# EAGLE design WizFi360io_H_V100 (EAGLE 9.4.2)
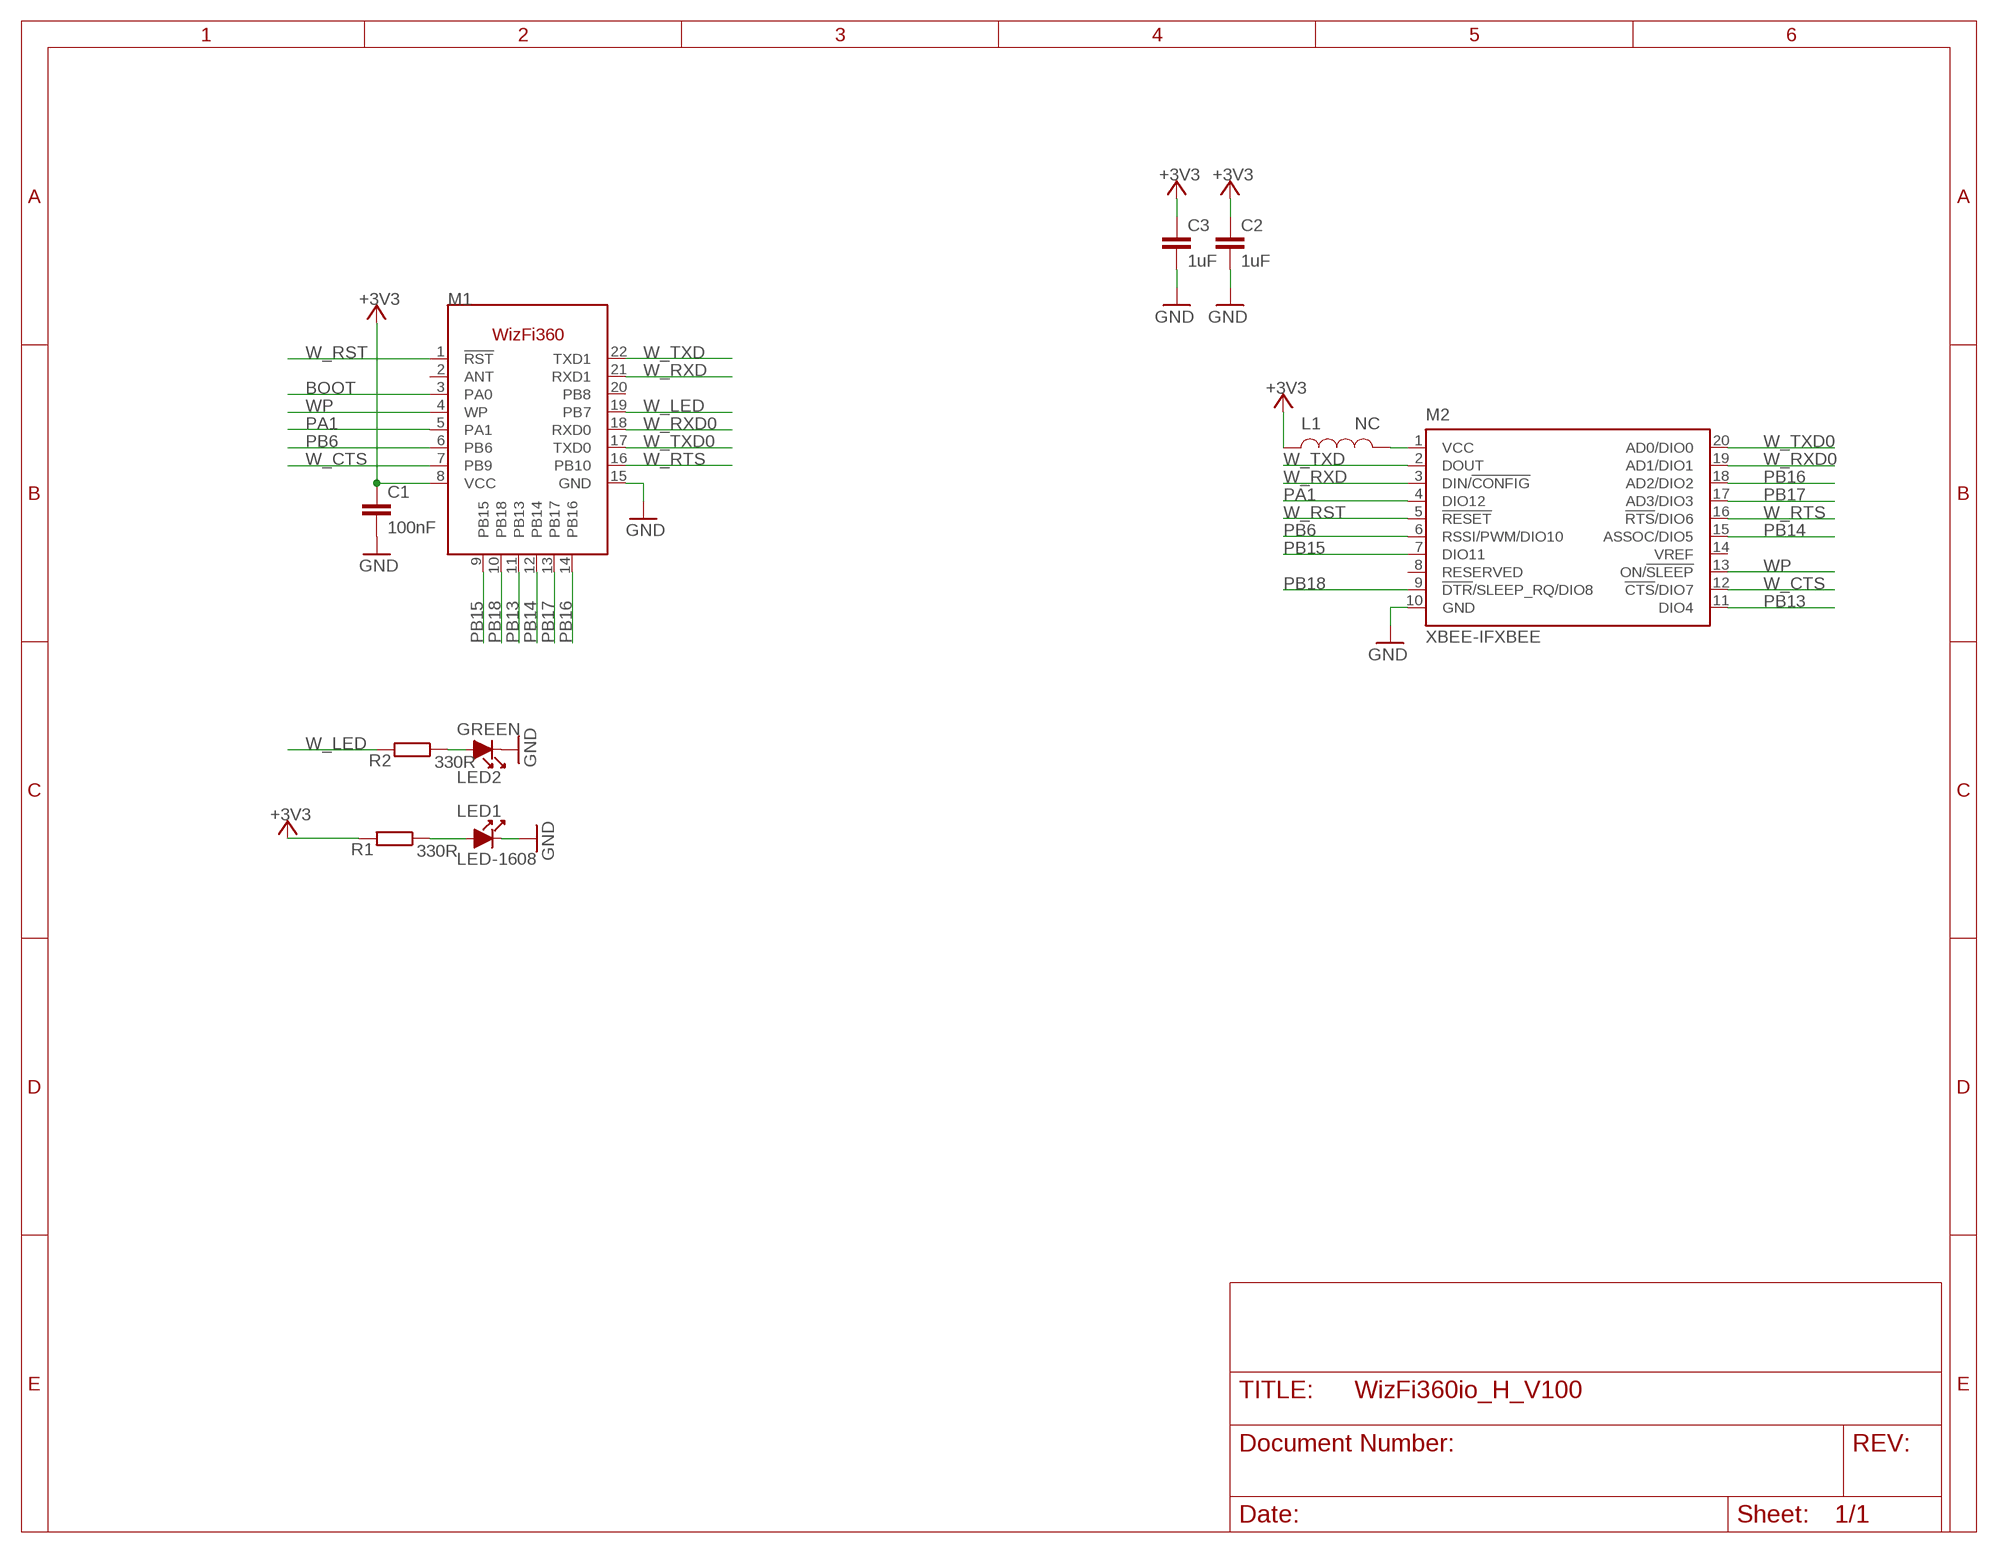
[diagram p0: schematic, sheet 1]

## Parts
C1  100nF  0142_10NF_0603  [C0603-ROUND@1]
C2  1uF  0142_10NF_0603  [C0603-ROUND@1]
C3  1uF  0142_10NF_0603  [C0603-ROUND@1]
L1  NC  L-1608  [L-1608]
LED1  LED-1608  [LED-1608]
LED2  GREEN  LED-1608  [LED-1608]
M1  WIZFI360  [WIZFI360]
M2  XBEE-IFXBEE  [XBEE-IF]
R1  330R  0028_CR0603JW103L  [R0603-ROUND]
R2  330R  0028_CR0603JW103L  [R0603-ROUND]

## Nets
+3V3 [power]: C1.1 C2.1 C3.1 L1.1 M1.8(VCC) R1.2
BOOT: M1.3(PA0)
GND: C1.2 C2.2 C3.2 LED1.K LED2.K M1.15(GND) M2.10(GND)
N$1: L1.P$2 M2.1(VCC)
N$7: LED1.A R1.1
N$17: LED2.A R2.1
PA1: M1.5(PA1) M2.4(DIO12)
PB6: M1.6(PB6) M2.6(RSSI/PWM/DIO10)
PB13: M1.11(PB13) M2.11(DIO4)
PB14: M1.12(PB14) M2.15(ASSOC/DIO5)
PB15: M1.9(PB15) M2.7(DIO11)
PB16: M1.14(PB16) M2.18(AD2/DIO2)
PB17: M1.13(PB17) M2.17(AD3/DIO3)
PB18: M1.10(PB18) M2.9(!DTR!/SLEEP_RQ/DIO8)
W_CTS: M1.7(PB9) M2.12(!CTS!/DIO7)
W_LED: M1.19(PB7) R2.2
W_RST: M1.1(!RST!) M2.5(!RESET)
W_RTS: M1.16(PB10) M2.16(!RTS!/DIO6)
W_RXD: M1.21(RXD1) M2.3(DIN/!CONFIG)
W_RXD0: M1.18(RXD0) M2.19(AD1/DIO1)
W_TXD: M1.22(TXD1) M2.2(DOUT)
W_TXD0: M1.17(TXD0) M2.20(AD0/DIO0)
WP: M1.4(WP) M2.13(ON/!SLEEP)
Unconnected: M1.2(ANT) M1.20(PB8) M2.8(RESERVED) M2.14(VREF)

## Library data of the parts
C1-C3 = Condensatori:0142_10NF_0603: 10nF 0603; CASE: 0603; MONTHLY_USAGE: _____; PART_NUMBER: 10nF_0603; PRICE: _____; SUPPLIER: _____; TYPE: Condensatori; VALUE: 10nF
L1 = INDUCTOR:L-1608
LED1 LED2 = DIODE:LED-1608
M1 = WIZnet:WIZFI360
M2 = xbee:XBEE-IF
R1 R2 = Resistenze:0028_CR0603JW103L: 10K 0603; CASE: 0603; MONTHLY_USAGE: _____; PART_NUMBER: CR0603JW103L; PRICE: _____; SUPPLIER: _____; TYPE: Resistenze; VALUE: 10k

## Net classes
0 default: width 0.203 mm, drill 0.008 mm, clearance 0.127 mm
1 power: width 0.305 mm, drill 0.3 mm, clearance 0.203 mm

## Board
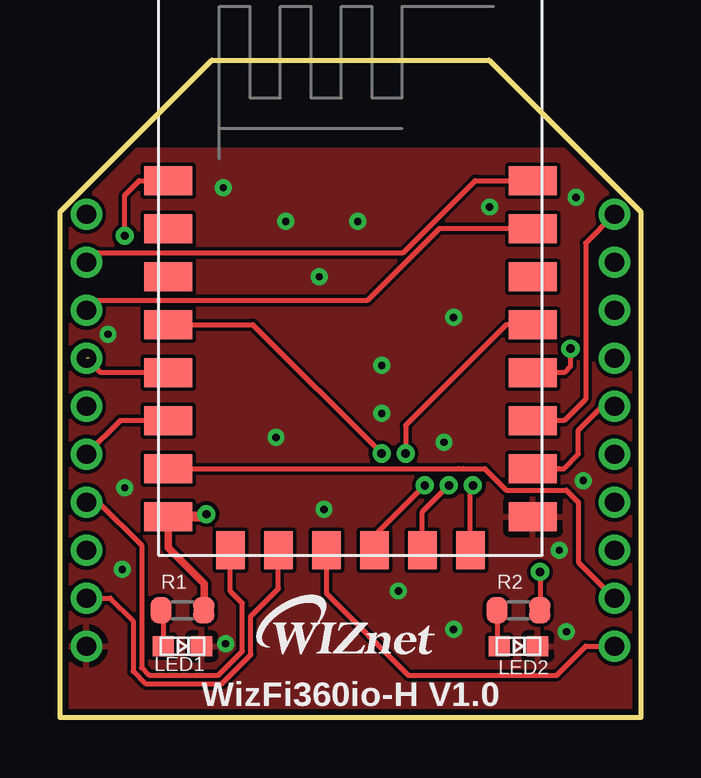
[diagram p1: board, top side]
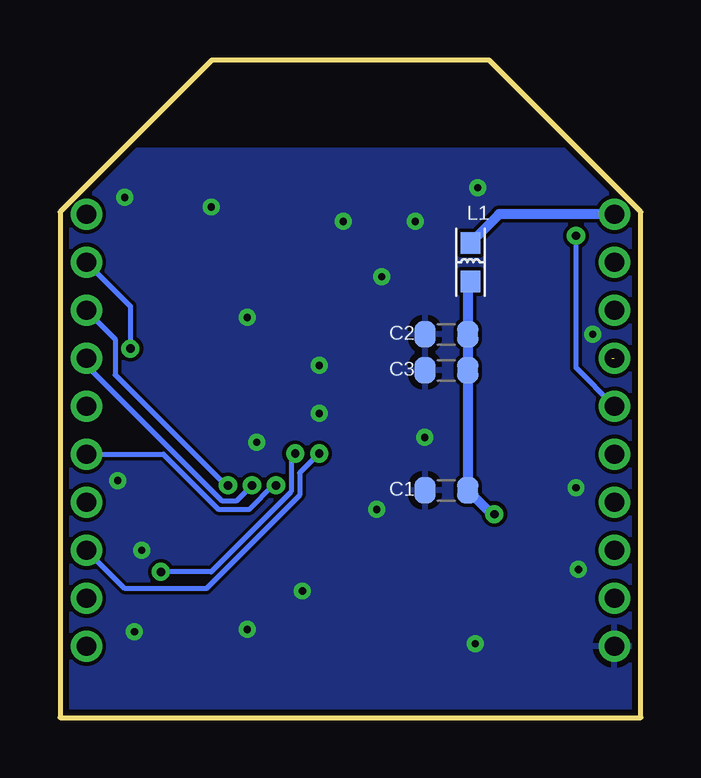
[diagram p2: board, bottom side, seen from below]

Size 24.2 x 27.4 mm. Coordinates in mm from the lower left corner, seen from the top.
Copper layers (1*16): Top 0.035mm / dielectric 1.5mm / Bottom 0.035mm
Design rules "default *": minimum track width 6mil, minimum drill 0.35mm, track to track 6mil, track to pad 6mil, pad to pad 6mil, via to via 6mil, smd to smd 6mil, copper to edge 10mil, drill to drill 10mil, minimum pad ring 10mil, minimum via ring 8mil, stop-mask expansion 4mil, vias tented up to drill 15mil, thermal gap 10mil

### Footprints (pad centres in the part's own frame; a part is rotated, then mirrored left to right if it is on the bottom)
C0603-ROUND@1 = smd 0.898 x 1.1: 1 -0.889,0; 2 0.889,0
L-1608 = smd 0.89 x 0.82: 1 -0.8,0; P$2 0.8,0
LED-1608 = smd 0.89 x 0.82: A -0.8,0; K 0.8,0
WIZFI360 = smd 2 x 1.2: 1 -7.6,3.6; 2 -7.6,1.6; 3 -7.6,-0.4; 4 -7.6,-2.4; 5 -7.6,-4.4; 6 -7.6,-6.4; 7 -7.6,-8.4; 8 -7.6,-10.4; 15 7.6,-10.4; 16 7.6,-8.4; 17 7.6,-6.4; 18 7.6,-4.4; 19 7.6,-2.4; 20 7.6,-0.4; 21 7.6,1.6; 22 7.6,3.6 | smd 1.2 x 1.6: 9 -5,-11.8; 10 -3,-11.8; 11 -1,-11.8; 12 1,-11.8; 13 3,-11.8; 14 5,-11.8
XBEE-IF = drill 0.8 pad 1.27: 1 -11,9; 2 -11,7; 3 -11,5; 4 -11,3; 5 -11,1; 6 -11,-1; 7 -11,-3; 8 -11,-5; 9 -11,-7; 10 -11,-9; 11 11,-9; 12 11,-7; 13 11,-5; 14 11,-3; 15 11,-1; 16 11,1; 17 11,3; 18 11,5; 19 11,7; 20 11,9
R0603-ROUND = smd 0.898 x 1.1: 1 -0.889,0; 2 0.889,0

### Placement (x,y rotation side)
C1  8.1,9.47 180 bottom
C2  8.1,15.97 180 bottom
C3  8.1,14.47 180 bottom
L1  7.1,18.98 90 bottom
LED1  5.1,2.97 0 top
LED2  19.1,2.97 0 top
M1  12.1,18.77 0 top
M2  12.1,11.97 0 top
R1  5.1,4.47 0 top
R2  19.1,4.47 0 top
U$1  [WIZNET3-LOGO]  8,2.62 0 top

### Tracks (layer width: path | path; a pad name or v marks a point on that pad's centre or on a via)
+3V3  (via drill 0.35)
  Top 0.305: M1.8 4.5,7.07 6,5.57 R1.2
  Top 0.406: v6.1,8.47 6,8.38 M1.8
  Bottom 0.406: L1.1 7.21,18.06 C2.1 C3.1 C1.1 6.21,8.47 v6.1,8.47
GND  (via drill 0.3)
  other vias: 14.1,5.27 6.9,3.07 20.8,6.97 21.1,3.57 13.4,12.67 16,11.47 9,11.67 10.8,18.38 17.9,21.27 21.5,21.67 6.8,22.08 2.7,9.57 2.6,6.17 11,8.67 13.4,14.67 16.4,16.67 12.4,20.67 9.4,20.67 16.4,3.67 21.8,9.88 2,15.97
  pour Top: -0.9,-1.03 25.1,-1.03 25.1,27.98 -0.9,27.98
  pour Bottom: -1.9,-2.03 26.1,-2.03 26.1,28.98 -1.9,28.98
N$1
  Bottom 0.406: M2.1 5.9,20.98 L1.P$2
N$7
  Top 0.203: R1.1 4.3,4.39 LED1.A
N$17
  Top 0.203: R2.1 18.21,3.06 LED2.A
PA1  (1 unrouted)
  Top 0.203: M1.5 1.7,14.38 1.22,14.86 1.22,14.97
PB6
  Top 0.203: M1.6 2.5,12.38 M2.6
PB13
  Top 0.203: M1.11 11.1,5.17 14.5,1.77 20.7,1.77 21.9,2.97 M2.11
PB14  (via drill 0.35)
  Top 0.203: M1.12 13.1,7.57 v15.2,9.67
  Bottom 0.203: M2.15 19.9,10.97 17.61,8.69 16.29,8.69 15.31,9.67 v15.2,9.67
PB15
  Top 0.203: M2.7 1.6,8.97 3.4,7.17 3.4,2.07 3.7,1.77 6.6,1.77 7.6,2.77 7.6,4.77 7.1,5.27 M1.9
PB16  (via drill 0.35)
  Top 0.203: M1.14 17.1,9.57 v17.2,9.67
  Bottom 0.203: M2.18 21.9,15.78 21.9,14.28 17.3,9.67 v17.2,9.67
PB17  (via drill 0.35)
  Top 0.203: M1.13 15.1,8.57 v16.2,9.67
  Bottom 0.203: M2.17 23.1,14.68 17.46,9.04 16.83,9.04 v16.2,9.67
PB18
  Top 0.203: M2.9 2.1,4.97 3.04,4.03 3.04,1.93 3.55,1.42 6.75,1.42 7.96,2.63 7.96,4.23 9.1,5.38 M1.10
W_CTS
  Top 0.203: M1.7 16.6,10.38 16.8,10.38 17.7,10.38 18.6,9.47 21.1,9.47 21.6,8.97 21.6,6.47 M2.12
W_LED  (via drill 0.35)
  Top 0.203: M1.19 18.6,16.38 14.4,12.17 v14.4,11.01 | v20,6.07 R2.2
  Bottom 0.203: v14.4,11.01 14.57,10.84 14.57,9.41 17.91,6.07 v20,6.07
W_RST  (via drill 0.35)
  Top 0.203: v2.7,20.08 2.7,21.77 3.3,22.38 M1.1
  Bottom 0.203: M2.5 2.7,14.57 v2.7,20.08
W_RTS
  Top 0.203: 20.8,10.38 M1.16 21,10.38 21.6,10.97 21.6,11.97 22.6,12.97 M2.16
W_RXD
  Top 0.203: M2.3 1.5,17.38 12.8,17.38 15.8,20.38 M1.21
W_RXD0  (via drill 0.35)
  Top 0.203: v21.27,15.38 21.27,14.64 21,14.38 M1.18
  Bottom 0.203: M2.19 21.27,17.14 v21.27,15.38
W_TXD
  Top 0.203: M1.22 17.3,22.38 14.3,19.38 1.5,19.38 M2.2
W_TXD0
  Top 0.203: M2.20 21.9,19.77 21.9,13.28 21,12.38 M1.17
WP  (via drill 0.35)
  Top 0.203: M1.4 8.03,16.38 v13.4,11.01
  Bottom 0.203: v13.4,11.01 14.21,10.2 14.21,9.27 18.1,5.38 21.5,5.38 M2.13

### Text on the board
tNames: WizFi360io-H V1.0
